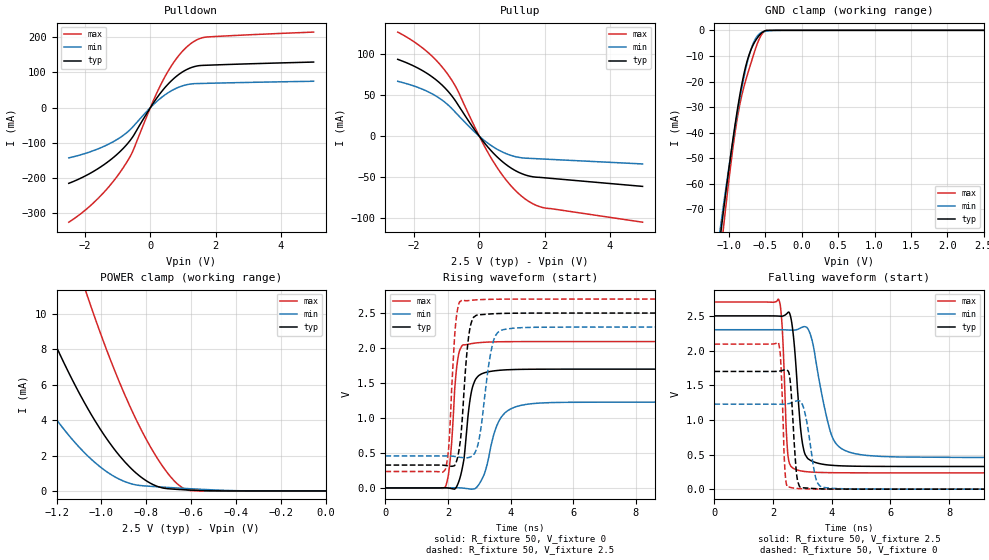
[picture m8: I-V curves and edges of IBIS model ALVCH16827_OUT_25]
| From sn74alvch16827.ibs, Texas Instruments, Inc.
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[Model]   ALVCH16827_OUT_25
Model_type  3-state
Enable   Active-Low
Vref =   0
Rref =   500
Cref =   30p
Vmeas =   1.25
| variable   typ   min   max
C_comp   4.10pF   3.64pF   4.32pF
| C_pullup   5.27pF   4.50pF   5.83pF
| C_pulldown   8.61pF   4.78pF   12.54pF
| C_tri-state   4.10pF   3.64pF   4.32pF
[Temperature Range]   40   100   -40
| Ambient temperature   25   85   -40
[Voltage range]   2.5   2.3   2.7
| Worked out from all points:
|   slope of the pulldown table from 0 to 0.375 V, typ, clamps not added: 7.66 ohm
|   slope of the pullup table from 0 to 0.375 V, typ, clamps not added: 20.6 ohm
|   GND clamp passes 1 mA (typ) near -0.55 V on its own axis
|   POWER clamp passes 1 mA (typ) near -0.84 V on its own axis
|   rising waveform, R_fixture 50, V_fixture 0: 20-80 % time 260ps typ, 466ps min, 193ps max; typ from 0 V to 1.7 V
|   falling waveform, R_fixture 50, V_fixture 2.5: 20-80 % time 242ps typ, 528ps min, 139ps max; typ from 2.5 V to 0.327 V
|   rising waveform, R_fixture 50, V_fixture 2.5: 20-80 % time 219ps typ, 324ps min, 174ps max; typ from 0.327 V to 2.5 V
|   falling waveform, R_fixture 50, V_fixture 0: 20-80 % time 152ps typ, 268ps min, 105ps max; typ from 1.7 V to 0 V
[GND Clamp]
| ALVCH16827_OUT_25
|   Voltage   I(typ)   I(min)   I(max)
-2.5V     -448.7mA   -408mA     -511.8mA
-1.12V    -80.81mA   -77.55mA   -88.84mA
-1.1V     -76.16mA   -73.37mA   -83.51mA
-1.08V    -71.57mA   -69.24mA   -78.26mA
-1.065V   -68.16mA   -66.17mA   -74.37mA
-985mV    -50.67mA   -50.33mA   -54.68mA
-910mV    -35.66mA   -36.52mA   -38.71mA
-800mV    -17.73mA   -19.03mA   -22.63mA
-685mV    -6.713mA   -6.416mA   -11.59mA
-555mV    -1.142mA   -838.4uA   -1.794mA
-480mV    -38.26uA   -264.2uA   -15.01uA
2.5V      1.191nA    103.3nA    39.45pA
[POWER Clamp]
| ALVCH16827_OUT_25
|   Voltage   I(typ)   I(min)   I(max)
-2.5V     62.78mA    42.4mA     93.4mA
-1.535V   19.08mA    11.24mA    32.91mA
-1.515V   18.34mA    10.73mA    31.84mA
-1.295V   10.9mA     5.78mA     20.85mA
-1.165V   7.185mA    3.45mA     15.09mA
-1.06V    4.638mA    1.967mA    10.93mA
-950mV    2.483mA    868.6uA    7.093mA
-845mV    1.005mA    337.4uA    4.026mA
-745mV    230.8uA    229.2uA    1.729mA
-655mV    82.47uA    160.2uA    326.5uA
-600mV    45.53uA    121.3uA    16.21uA
-31.15fV  1.191nA    59.92nA    46.96pA
[Pulldown]
| ALVCH16827_OUT_25
|   Voltage   I(typ)   I(min)   I(max)
-2.5V     -214.5mA   -142.4mA   -324.7mA
-1.625V   -174.1mA   -117.7mA   -259.4mA
-1.225V   -148.2mA   -100.9mA   -219.1mA
-870mV    -119.2mA   -81.23mA   -175.5mA
-550mV    -84.06mA   -55.7mA    -125.8mA
75mV      10.83mA    7.022mA    16.48mA
430mV     55.09mA    35.04mA    84.84mA
820mV     90.47mA    55.98mA    141.7mA
1.215V    112.2mA    66.71mA    179.9mA
1.465V    118.6mA    68.28mA    193.9mA
1.72V     120.2mA    68.88mA    200.2mA
5V        129.2mA    74.77mA    214.1mA
[Pullup]
| ALVCH16827_OUT_25
|   Voltage   I(typ)   I(min)   I(max)
-2.5V     93.89mA    67.09mA    127.2mA
-1.675V   78.56mA    56.27mA    105.7mA
-1.335V   69.15mA    49.28mA    93.27mA
-1.035V   58.23mA    40.89mA    79.35mA
-685mV    40.38mA    27.22mA    57.59mA
15mV      -812.9uA   -531.7uA   -1.2mA
420mV     -20.15mA   -12.8mA    -30.36mA
885mV     -36.42mA   -22.17mA   -56.52mA
1.355V    -46.47mA   -26.53mA   -75.01mA
1.67V     -49.6mA    -27.19mA   -82.95mA
1.985V    -50.63mA   -27.82mA   -87.32mA
5V        -61.14mA   -33.76mA   -104.8mA
[Ramp]
| ALVCH16827_OUT_25
| variable   typ   min   max
dV/dt_r   1.03/2.76E-10   0.75/4.74E-10   1.26/2.09E-10
dV/dt_f   1.34/2.59E-10   1.13/5.39E-10   1.50/1.50E-10
R_load = 50
[Rising Waveform]
| ALVCH16827_OUT_25
R_fixture =   50
C_fixture =   0
L_fixture =   0
V_fixture =   0
V_fixture_min = 0
V_fixture_max = 0
|   Time   V(typ)   V(min)   V(max)
0s        298.3pV    1.147nV    220.6pV
1.915ns   3.258mV    123.3uV    15.86mV
2.06ns    -4.314mV   1.308mV    365.7mV
2.23ns    -8.998mV   2.913mV    1.507V
2.35ns    99.55mV    2.184mV    1.934V
2.735ns   1.347V     -16.26mV   2.062V
2.98ns    1.606V     45.43mV    2.076V
3.72ns    1.685V     1.024V     2.09V
4.96ns    1.698V     1.214V     2.092V
50ns      1.698V     1.227V     2.092V
[Falling Waveform]
| ALVCH16827_OUT_25
R_fixture =   50
C_fixture =   0
L_fixture =   0
V_fixture =   2.5
V_fixture_min = 2.3
V_fixture_max = 2.7
|   Time   V(typ)   V(min)   V(max)
0s        2.5V       2.3V       2.7V
2.19ns    2.497V     2.3V       2.736V
2.305ns   2.495V     2.3V       2.367V
2.52ns    2.554V     2.296V     443.7mV
2.675ns   2.275V     2.294V     303.7mV
2.93ns    899.8mV    2.324V     264.7mV
3.085ns   506.8mV    2.344V     254.4mV
4.055ns   342.5mV    718.1mV    237.5mV
5.225ns   329.2mV    485.2mV    235.5mV
50ns      327.2mV    457.5mV    235.2mV
[Rising Waveform]
| ALVCH16827_OUT_25
R_fixture =   50
C_fixture =   0
L_fixture =   0
V_fixture =   2.5
V_fixture_min = 2.3
V_fixture_max = 2.7
|   Time   V(typ)   V(min)   V(max)
0s        327.2mV    457.5mV    235.2mV
1.915ns   322mV      458.2mV    266mV
2.025ns   313.7mV    457.6mV    602.2mV
2.25ns    356.1mV    448.4mV    2.374V
2.465ns   1.056V     433.9mV    2.689V
2.63ns    2.055V     432mV      2.677V
2.795ns   2.425V     467.3mV    2.685V
3.46ns    2.49V      2.113V     2.697V
4.1ns     2.498V     2.284V     2.7V
50ns      2.5V       2.3V       2.7V
[Falling Waveform]
| ALVCH16827_OUT_25
R_fixture =   50
C_fixture =   0
L_fixture =   0
V_fixture =   0
V_fixture_min = 0
V_fixture_max = 0
|   Time   V(typ)   V(min)   V(max)
0s        1.698V     1.227V     2.092V
2.175ns   1.701V     1.225V     2.118V
2.26ns    1.707V     1.225V     1.839V
2.435ns   1.723V     1.228V     116.4mV
2.585ns   1.55V      1.24V      26.01mV
2.785ns   278.2mV    1.271V     11.1mV
3.065ns   18.52mV    1.135V     4.971mV
3.5ns     6.654mV    102mV      1.757mV
4.08ns    1.842mV    11.09mV    493.5uV
50ns      110.7nV    1.86nV     10.09nV
